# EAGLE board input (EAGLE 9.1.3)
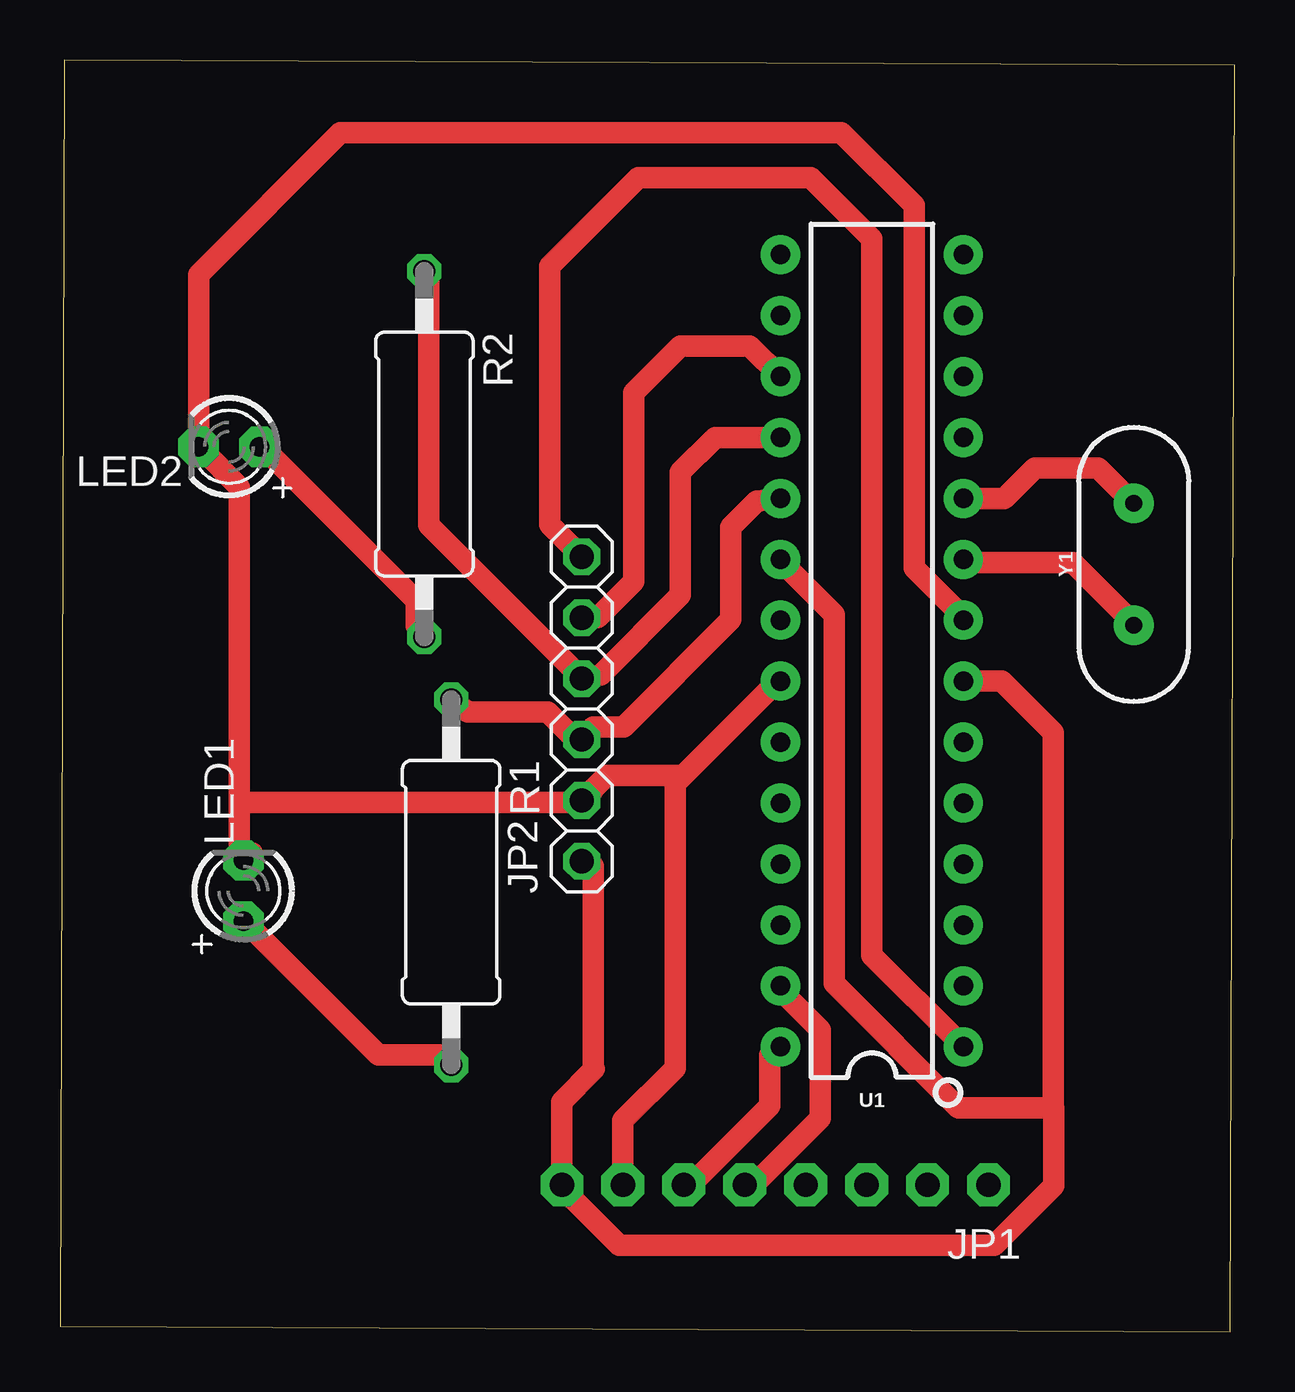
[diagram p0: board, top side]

Size 48.95 x 53 mm. Coordinates in mm from the lower left corner, seen from the top.
Outline: 0,0.22 48.77,0 48.95,52.78 0.18,53 0,0.22
Copper layers (1*16): Top 0.035mm / dielectric 1.5mm / Bottom 0.035mm
Design rules "default *": minimum track width 0.9mm, minimum drill 0.35mm, track to track 6mil, track to pad 6mil, pad to pad 6mil, via to via 6mil, smd to smd 6mil, copper to edge 40mil, drill to drill 6mil, minimum pad ring 10mil, minimum via ring 8mil, stop-mask expansion 4mil, vias tented up to drill 0mil, thermal gap 10mil

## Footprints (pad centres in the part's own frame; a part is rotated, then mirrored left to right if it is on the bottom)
1X08-CLEANBIG = drill 1.016 pad 1.778 octagon: 1 -8.89,0; 2 -6.35,0; 3 -3.81,0; 4 -1.27,0; 5 1.27,0; 6 3.81,0; 7 6.35,0; 8 8.89,0
1X06 = drill 1.016 octagon: 1 -6.35,0; 2 -3.81,0; 3 -1.27,0; 4 1.27,0; 5 3.81,0; 6 6.35,0
LED3MM = drill 0.813 pad 1.676 octagon: A -1.27,0; K 1.27,0
0411/15 = drill 0.914 octagon: 1 -7.62,0; 2 7.62,0
DIP28 = drill 0.813 pad 1.626: 1 -16.51,-3.81; 2 -13.97,-3.81; 3 -11.43,-3.81; 4 -8.89,-3.81; 5 -6.35,-3.81; 6 -3.81,-3.81; 7 -1.27,-3.81; 8 1.27,-3.81; 9 3.81,-3.81; 10 6.35,-3.81; 11 8.89,-3.81; 12 11.43,-3.81; 13 13.97,-3.81; 14 16.51,-3.81; 15 16.51,3.81; 16 13.97,3.81; 17 11.43,3.81; 18 8.89,3.81; 19 6.35,3.81; 20 3.81,3.81; 21 1.27,3.81; 22 -1.27,3.81; 23 -3.81,3.81; 24 -6.35,3.81; 25 -8.89,3.81; 26 -11.43,3.81; 27 -13.97,3.81; 28 -16.51,3.81
HC49US = drill 0.7 pad 1.651: 1 -2.54,0; 2 2.54,0

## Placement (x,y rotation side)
JP1  [1X08-CLEANBIG]  29.8,6.12 180 top
JP2  [1X06]  21.74,25.95 90 top
LED1  [LED3MM]  7.64,18.37 90 top
LED2  [LED3MM]  7.04,36.88 180 top
R1  [0411/15]  16.3,18.73 270 top
R2  [0411/15]  15.18,36.58 270 top
U1  328P  [DIP28]  33.83,28.38 90 top
Y1  16MHz  [HC49US]  44.74,31.98 90 top

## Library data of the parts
JP1 JP2 LED1 LED2 R1 R2 = adafruit
U1 = SparkFun-IC-Microcontroller; PROD_ID: IC-09136
Y1 = SparkFun-Clocks; PROD_ID: XTAL-08181; SF_ID: COM-00536

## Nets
GND: JP1.7 JP2.2 LED1.K LED2.K U1.8 U1.22
N$1: U1.10 Y1.2
N$2: U1.9 Y1.1
N$3: JP2.3 R1.1 U1.19
N$4: JP2.4 R2.1 U1.18
N$5: LED2.A R2.2
N$6: LED1.A R1.2
N$7: JP2.5 U1.17
N$8: JP1.6 U1.28
N$9: JP1.5 U1.27
N$10: JP2.6 U1.1
VCC: JP1.8 JP2.1 U1.7 U1.20

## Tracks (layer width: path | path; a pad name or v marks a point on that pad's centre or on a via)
GND
  Top 0.9: 29.58,26.79 U1.22 29.58,26.79 | 8,19.95 LED1.K 7.48,19.95 7.48,22.05 | U1.8 37.47,29.94 35.59,31.83 35.59,46.96 32.56,49.98 11.69,49.98 5.77,44.07 LED2.K 5.9,36.78 7.48,35.2 7.48,22.05 | JP1.7 23.45,8.8 25.63,10.98 25.63,22.84 25.97,23.18 | 29.58,26.79 25.97,23.18 | 22.21,22.58 JP2.2 | 7.48,22.05 21.68,22.05 JP2.2 | JP2.2 22.77,23.18 25.97,23.18
N$1
  Top 0.9: Y1.2 43.27,35.99 40.62,35.99 39.35,34.73 U1.10
N$2
  Top 0.9: U1.9 38,32.05 42.21,32.05 44.31,29.94 Y1.1
N$3
  Top 0.9: U1.19 29.03,34.61 27.95,33.53 27.95,29.68 23.48,25.21 22.21,25.21 JP2.3 21.46,24.68 20.33,25.82 17,25.82 16.42,26.26 R1.1
N$4
  Top 0.9: R2.1 15.37,44.15 15.37,34.15 15.37,33.63 21.68,27.31 JP2.4 22.53,27.37 25.85,30.69 25.85,35.83 27.3,37.27 U1.18
N$5
  Top 0.9: R2.2 14.84,29.42 14.84,30.47 8.53,36.78 LED2.A
N$6
  Top 0.9: R1.2 15.9,11.52 13.26,11.52 8,16.79 LED1.A
N$7
  Top 0.9: U1.17 28.75,41.08 25.84,41.08 23.9,39.14 23.9,31.26 22.4,29.76 JP2.5
N$8
  Top 0.9: U1.28 29.58,11.52 29.58,9.42 26.42,6.26 JP1.6
N$9
  Top 0.9: U1.27 30.1,14.16 31.68,12.58 31.68,8.89 29.05,6.26 JP1.5
N$10
  Top 0.9: U1.1 37.47,12.05 33.83,15.69 33.83,45.55 31.29,48.1 24.09,48.1 20.41,44.41 20.41,33.63 JP2.6
VCC
  Top 0.9: 41.39,9.33 41.39,24.97 39.25,27.11 U1.7 | 41.39,9.33 41.42,9.33 41.42,6.09 38.92,3.59 23.31,3.59 21.16,5.74 JP1.8 20.91,9.59 22.27,10.94 22.21,11 22.21,19.42 JP2.1 | U1.20 30.1,32.05 32.25,29.9 32.25,14.51 37.43,9.33 40.63,9.33 41.39,9.33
